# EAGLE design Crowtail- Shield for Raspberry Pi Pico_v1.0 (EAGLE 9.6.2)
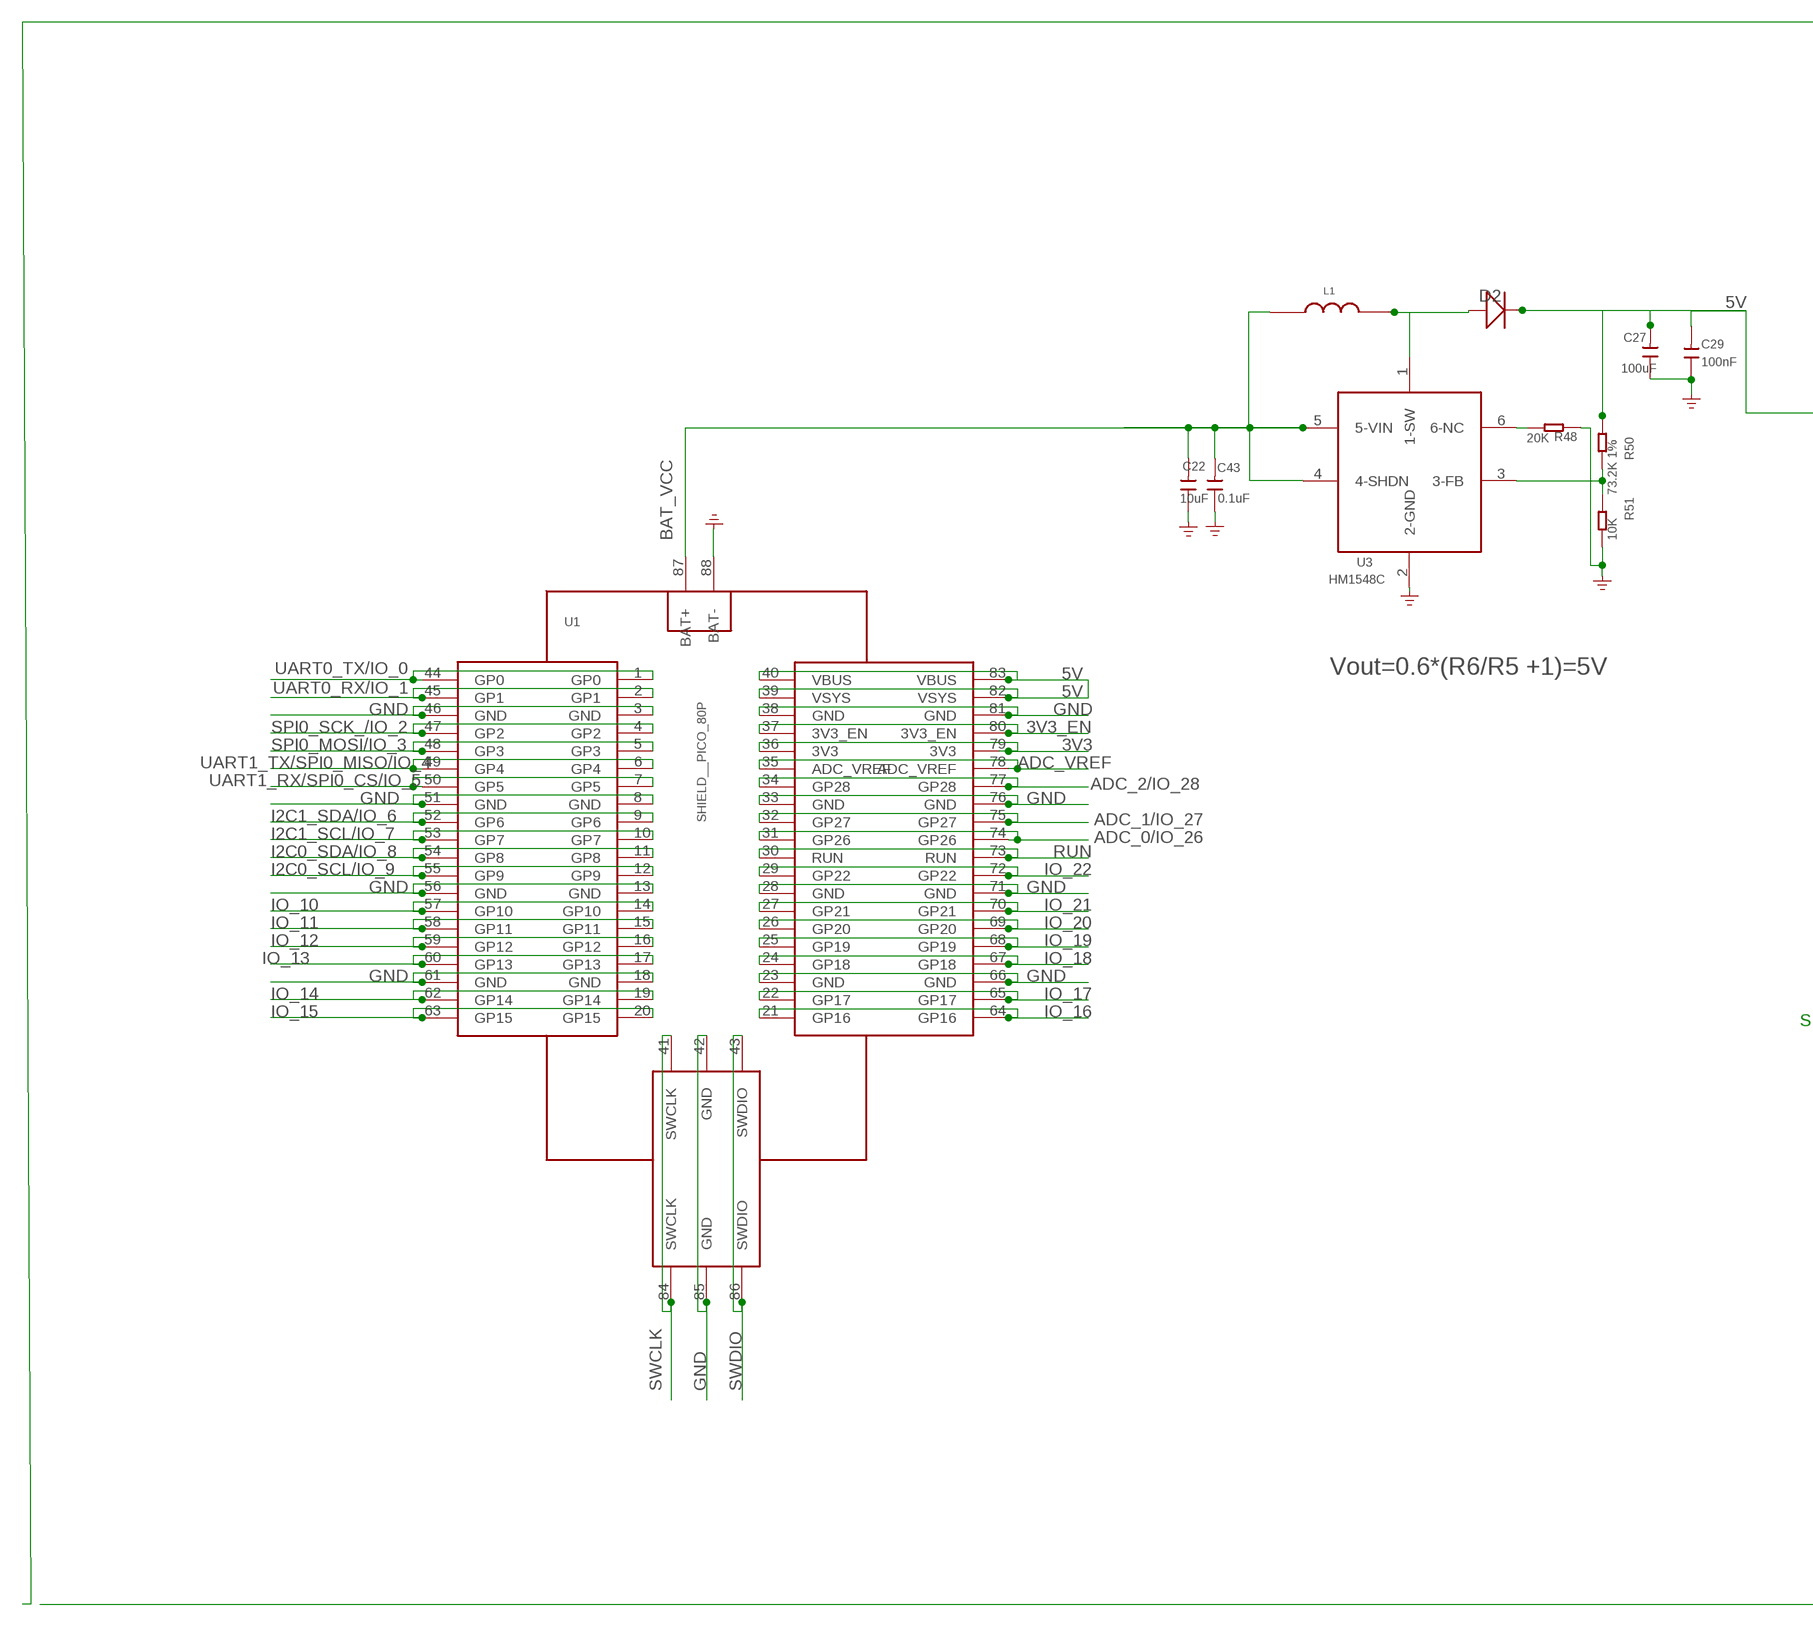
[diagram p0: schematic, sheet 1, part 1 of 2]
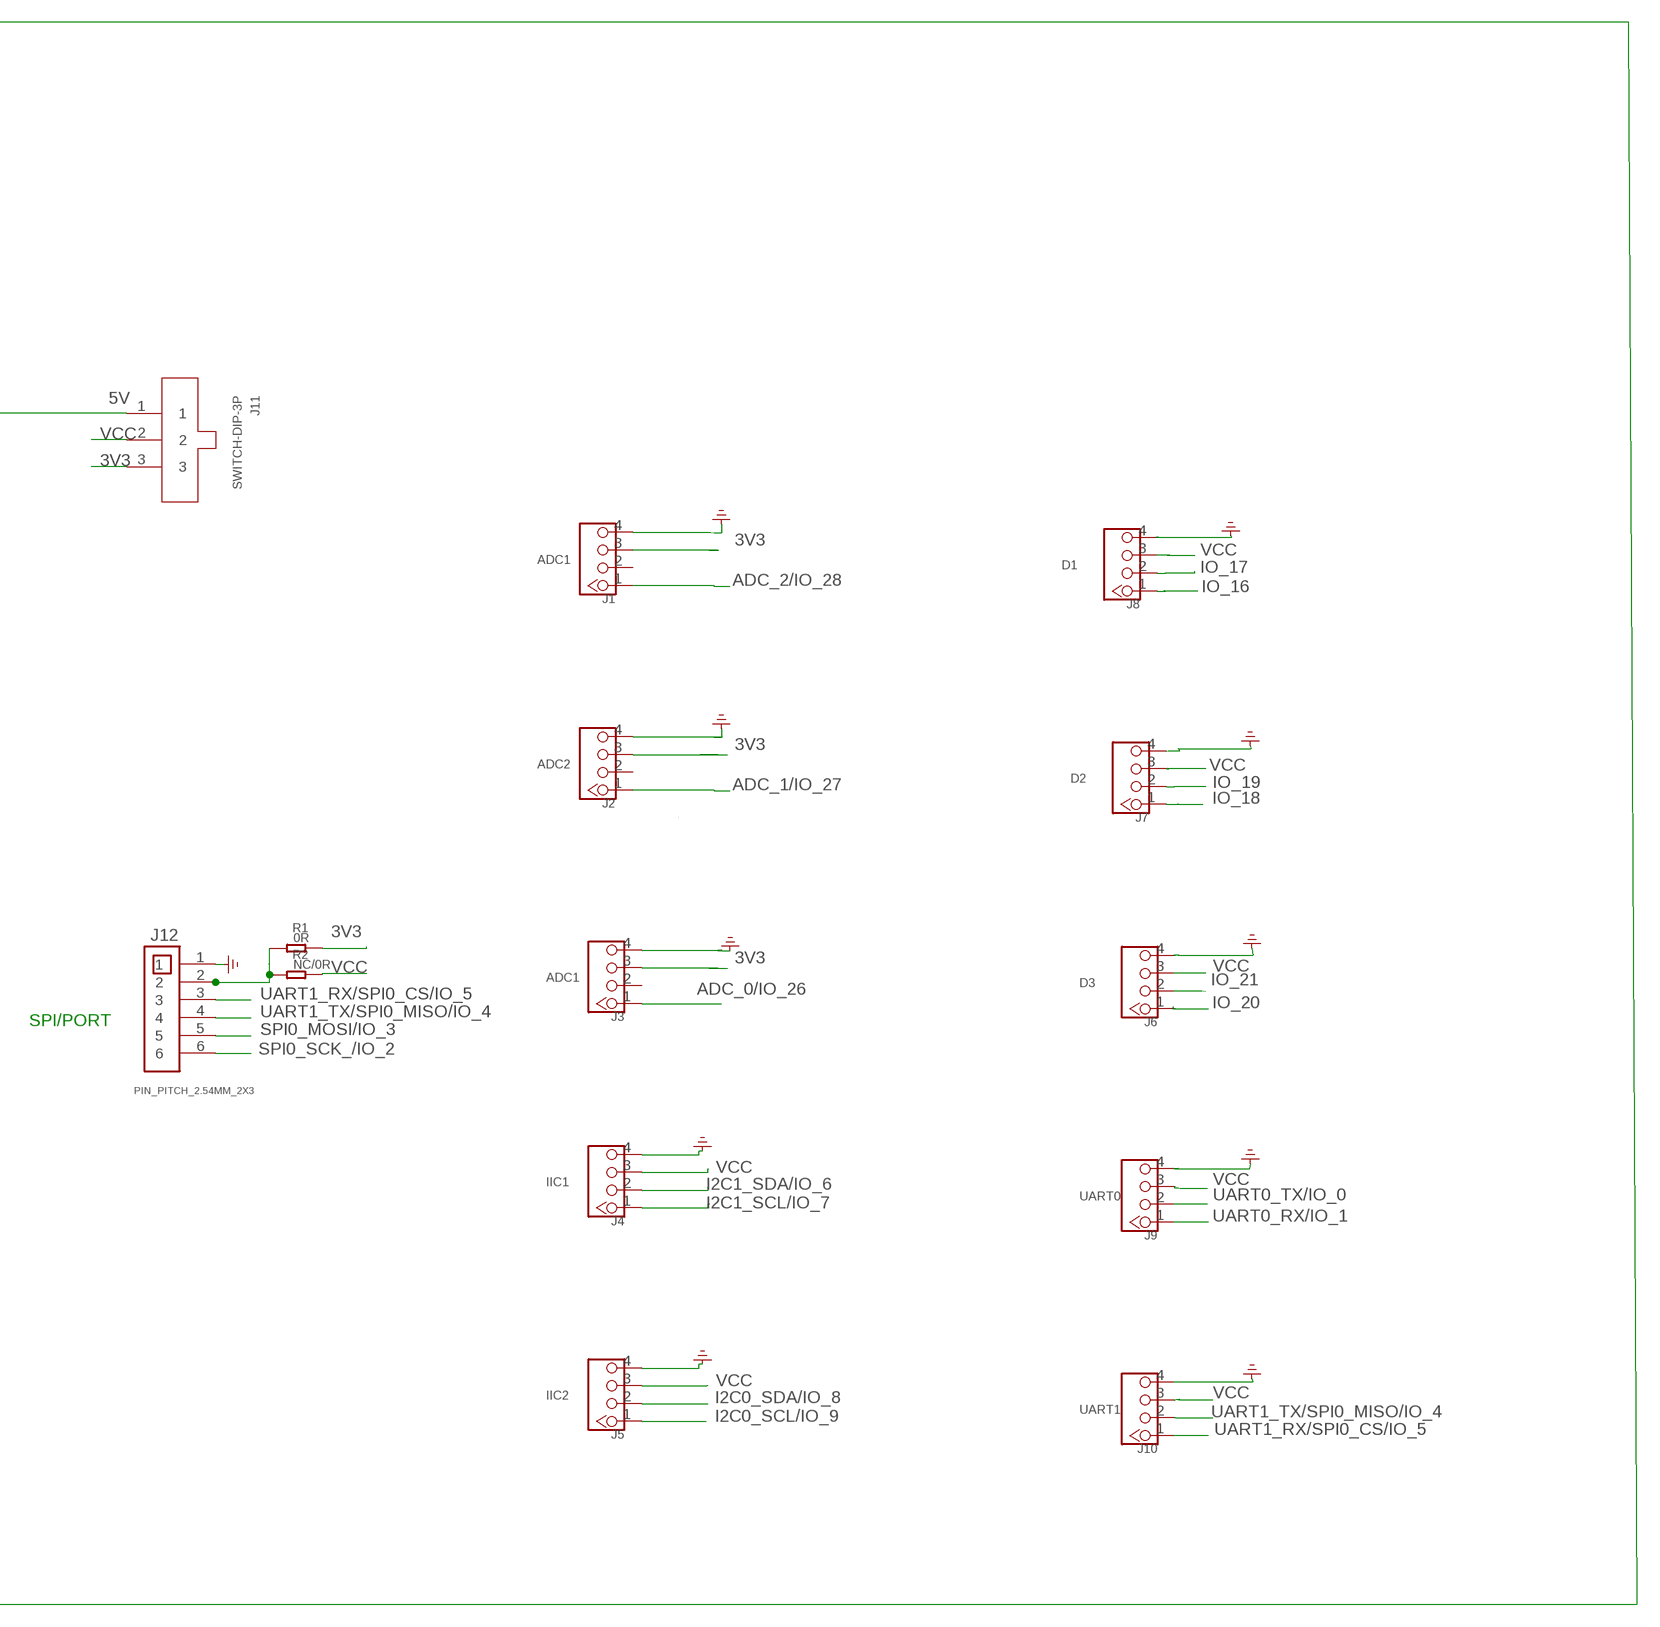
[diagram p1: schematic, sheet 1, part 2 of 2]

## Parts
C22  10uF  C0603  [0603]
C27  100uF  C0805  [0805]
C29  100nF  C0603  [0603]
C43  0.1uF  C0805  [0805]
D2  1N5819/S0D-123  D'1N4148-SMD'  [1206-1]
J1  ADC1  CONNECTOR_TWIG-4P-2.0-2.0  [CONNECTOR_4P-2.0]
J2  ADC2  CONNECTOR_TWIG-4P-2.0-2.0  [CONNECTOR_4P-2.0]
J3  ADC1  CONNECTOR_TWIG-4P-2.0-2.0  [CONNECTOR_4P-2.0]
J4  IIC1  CONNECTOR_TWIG-4P-2.0-2.0  [CONNECTOR_4P-2.0]
J5  IIC2  CONNECTOR_TWIG-4P-2.0-2.0  [CONNECTOR_4P-2.0]
J6  D3  CONNECTOR_TWIG-4P-2.0-2.0  [CONNECTOR_4P-2.0]
J7  D2  CONNECTOR_TWIG-4P-2.0-2.0  [CONNECTOR_4P-2.0]
J8  D1  CONNECTOR_TWIG-4P-2.0-2.0  [CONNECTOR_4P-2.0]
J9  UART0  CONNECTOR_TWIG-4P-2.0-2.0  [CONNECTOR_4P-2.0]
J10  UART1  CONNECTOR_TWIG-4P-2.0-2.0  [CONNECTOR_4P-2.0]
J11  SWITCH-DIP-3P  [SWITCH-DIP-3P]
J12  PIN_PITCH_2.54MM_2X3  [PIN6_PITCH_2.54MM_2X3]
L1  CD32_10uH  CD32_950MA  [CD32]
R1  0R  DISCRETE_R-0603  [DISCRETE_R0603]
R2  NC/0R  DISCRETE_R-0603  [DISCRETE_R0603]
R48  20K  DISCRETE_R-0603  [DISCRETE_R0603]
R50  73.2K 1%  DISCRETE_R-0603  [DISCRETE_R0603]
R51  10K  DISCRETE_R-0603  [DISCRETE_R0603]
U1  SHIELD__PICO_80P  [SHIELD__PICO_80P]
U3  HM1548C  HM1548/SOT23-6  [A_XBJ_SOT23-6]

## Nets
3V1: J12.2 R1.1 R2.1
3V3: J1.3 J2.3 J3.3 J11.3 R1.2 U1.36(3V3) U1.79(3V3)
3V3_EN: U1.37(3V3_EN) U1.80(3V3_EN)
5V: C27.2 C29.2 D2.C(-) J11.1 R50.1 U1.39(VSYS) U1.40(VBUS) U1.82(VSYS) U1.83(VBUS)
ADC_0/IO_26: J3.1 U1.31(GP26) U1.74(GP26)
ADC_1/IO_27: J2.1 U1.32(GP27) U1.75(GP27)
ADC_2/IO_28: J1.1 U1.34(GP28) U1.77(GP28)
ADC_VREF: U1.35(ADC_VREF) U1.78(ADC_VREF)
BAT_VCC: C22.2 C43.2 L1.1 U1.87(BAT+) U3.4(4-SHDN) U3.5(5-VIN)
GND: C22.1 C27.1 C29.1 C43.1 J1.4 J2.4 J3.4 J4.4 J5.4 J6.4 J7.4 J8.4 J9.4 J10.4 J12.1 R48.1 R51.2 U1.3(GND) U1.8(GND) U1.13(GND) U1.18(GND) U1.23(GND) U1.28(GND) U1.33(GND) U1.38(GND) U1.42(GND) U1.46(GND) U1.51(GND) U1.56(GND) U1.61(GND) U1.66(GND) U1.71(GND) U1.76(GND) U1.81(GND) U1.85(GND) U1.88(BAT-) U3.2(2-GND) ; supply symbol labelled GND_POWER
I2C0_SCL/IO_9: J5.1 U1.12(GP9) U1.55(GP9)
I2C0_SDA/IO_8: J5.2 U1.11(GP8) U1.54(GP8)
I2C1_SCL/IO_7: J4.1 U1.10(GP7) U1.53(GP7)
I2C1_SDA/IO_6: J4.2 U1.9(GP6) U1.52(GP6)
IO_10: U1.14(GP10) U1.57(GP10)
IO_11: U1.15(GP11) U1.58(GP11)
IO_12: U1.16(GP12) U1.59(GP12)
IO_13: U1.17(GP13) U1.60(GP13)
IO_14: U1.19(GP14) U1.62(GP14)
IO_15: U1.20(GP15) U1.63(GP15)
IO_16: J8.1 U1.21(GP16) U1.64(GP16)
IO_17: J8.2 U1.22(GP17) U1.65(GP17)
IO_18: J7.1 U1.24(GP18) U1.67(GP18)
IO_19: J7.2 U1.25(GP19) U1.68(GP19)
IO_20: J6.1 U1.26(GP20) U1.69(GP20)
IO_21: J6.2 U1.27(GP21) U1.70(GP21)
IO_22: U1.29(GP22) U1.72(GP22)
N$7: D2.A(+) L1.2 U3.1(1-SW)
N$24: R48.2 U3.6(6-NC)
N$30: R50.2 R51.1 U3.3(3-FB)
RUN: U1.30(RUN) U1.73(RUN)
SPI0_MOSI/IO_3: J12.5 U1.5(GP3) U1.48(GP3)
SPI0_SCK_/IO_2: J12.6 U1.4(GP2) U1.47(GP2)
SWCLK: U1.41(SWCLK) U1.84(SWCLK)
SWDIO: U1.43(SWDIO) U1.86(SWDIO)
UART0_RX/IO_1: J9.1 U1.2(GP1) U1.45(GP1)
UART0_TX/IO_0: J9.2 U1.1(GP0) U1.44(GP0)
UART1_RX/SPI0_CS/IO_5: J10.1 J12.3 U1.7(GP5) U1.50(GP5)
UART1_TX/SPI0_MISO/IO_4: J10.2 J12.4 U1.6(GP4) U1.49(GP4)
VCC: J4.3 J5.3 J6.3 J7.3 J8.3 J9.3 J10.3 J11.2 R2.2
Unconnected: J1.2 J2.2 J3.2

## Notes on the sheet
- Vout=0.6*(R6/R5 +1)=5V
- SPI/PORT

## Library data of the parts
C22 C29 = A_xbj:C0603
C27 C43 = A_xbj:C0805
D2 = Discrete:D*
J1-J10 = Crowtail_Shieldv0_1:CONNECTOR_TWIG-4P-2.0
J11 = Crowtail_Shieldv0_1:SWITCH-DIP-3P
J12 = PIN_PITCH_2.54MM:PIN_PITCH_2.54MM_2X3
L1 = CD54:CD32_950MA
R1 R2 R48 R50 R51 = Crowtail-_LED-V2.0-20190615-01:DISCRETE_R*
U1 = Crowtail_Shieldv0_1:SHIELD__PICO_80P
U3 = CrowBOT-V1.0-20220530库:HM1548/SOT23-6

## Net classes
0 default: width 0.203 mm, drill 0.305 mm, clearance 0.152 mm
3 usbvcc: width 0.203 mm, drill 0.305 mm, clearance 0.203 mm

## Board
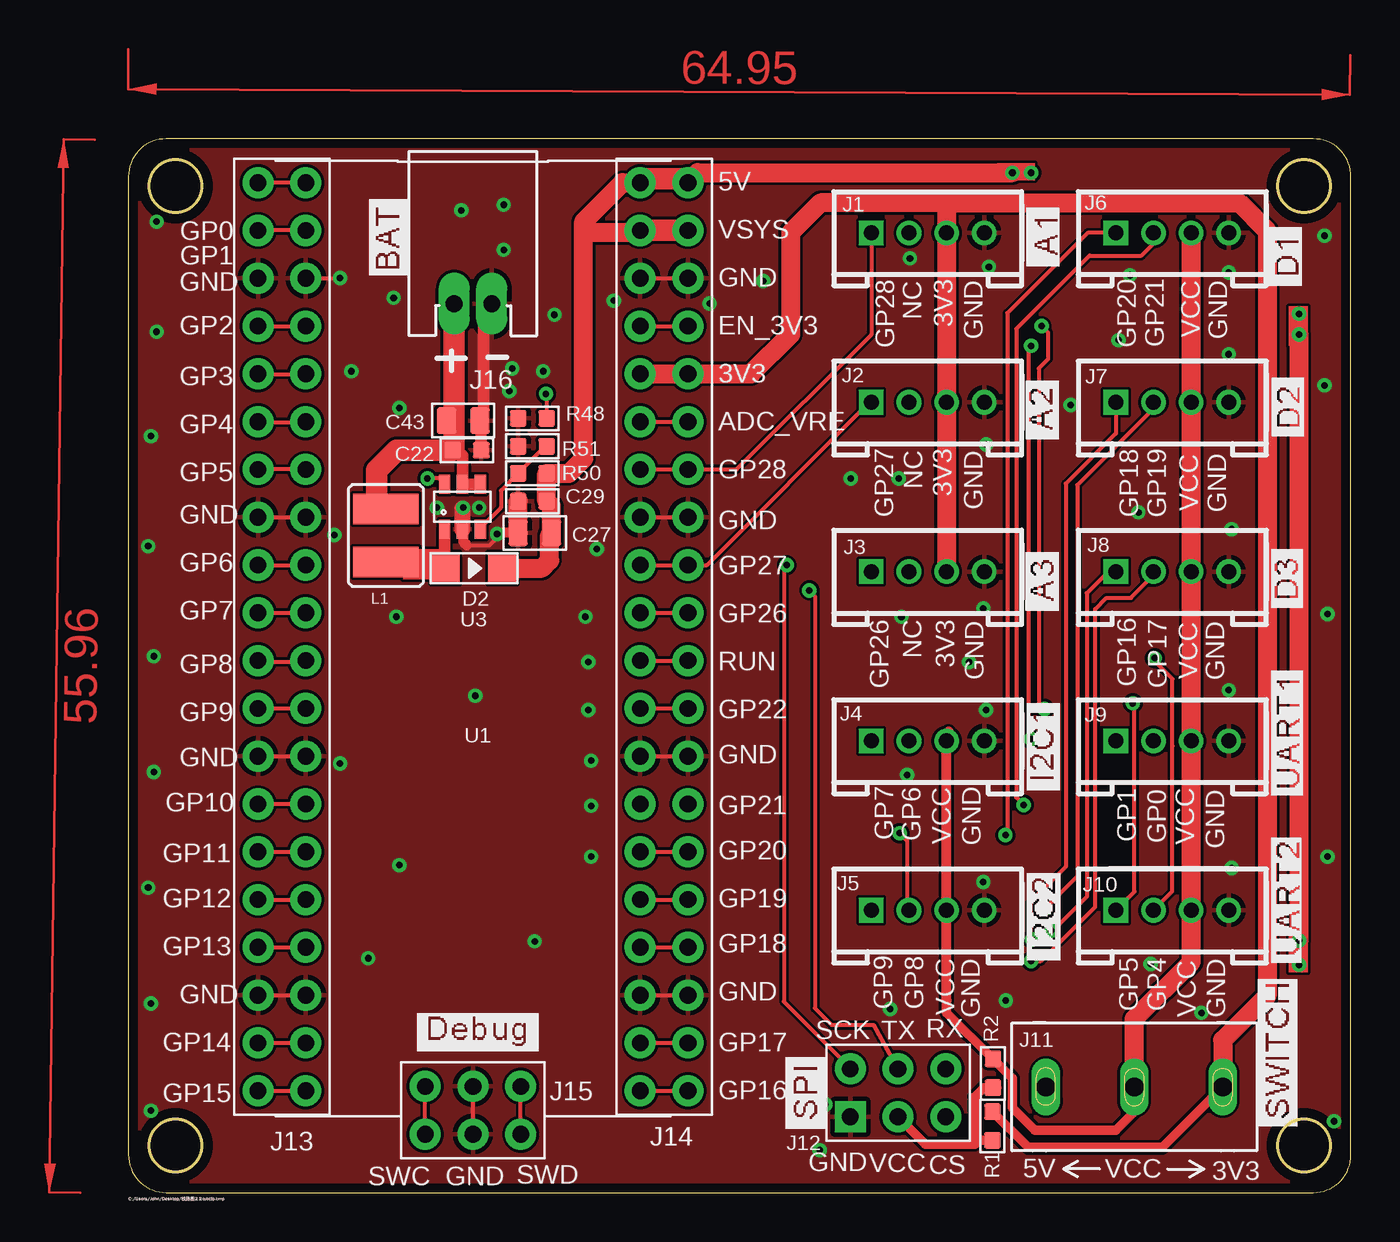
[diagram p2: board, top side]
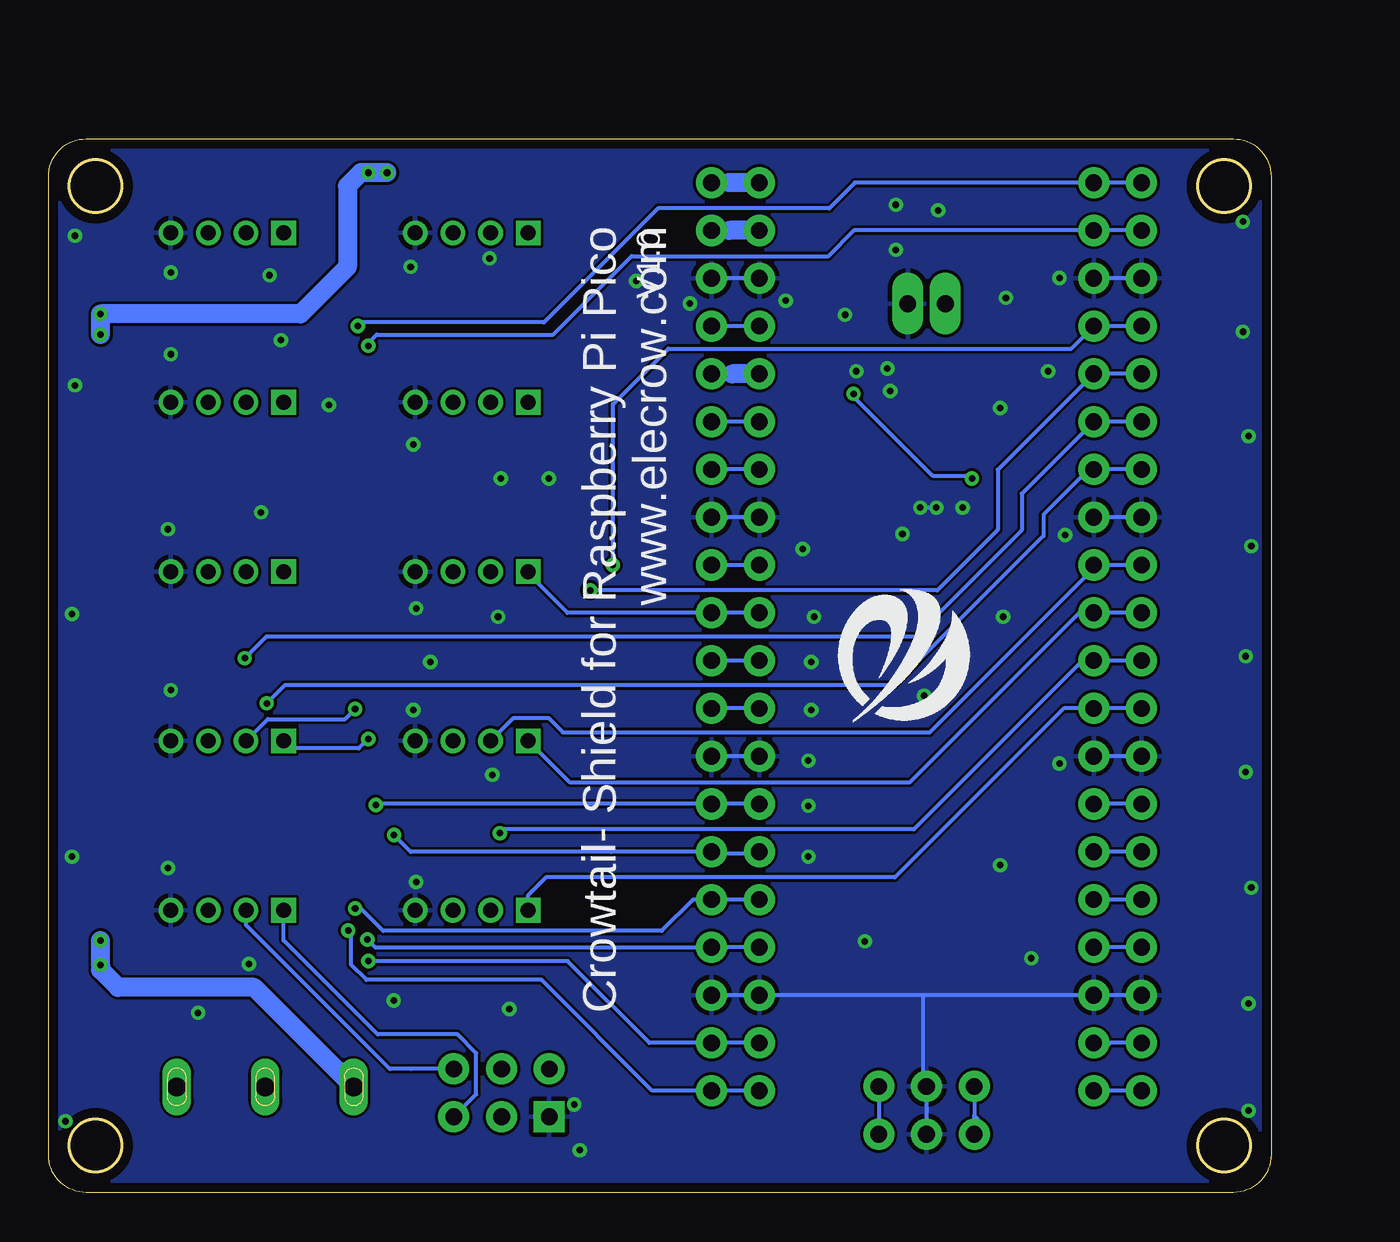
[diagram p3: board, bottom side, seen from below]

Size 65 x 56 mm. Coordinates in mm from the lower left corner, seen from the top.
Outline: 0,54 0,2 arc90 2,0 63,0 arc90 65,2 65,54 arc90 63,56 2,56 arc90 0,54
Outline: circle at 2.5,53.5 radius 1.4
Outline: circle at 2.5,2.5 radius 1.4
Outline: circle at 62.5,53.5 radius 1.4
Outline: circle at 62.5,2.5 radius 1.4
Copper layers (1*16): Top 0.035mm / dielectric 1.5mm / Bottom 0.035mm
Design rules "default *": minimum track width 6mil, minimum drill 0.35mm, track to track 6mil, track to pad 6mil, pad to pad 6mil, via to via 6mil, smd to smd 6mil, copper to edge 20mil, drill to drill 6mil, minimum pad ring 10mil, minimum via ring 8mil, stop-mask expansion 4mil, vias tented up to drill 20mil, thermal gap 10mil

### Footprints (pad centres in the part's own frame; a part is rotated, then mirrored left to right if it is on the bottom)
0603 = smd 0.889 x 0.889: 1 -0.762,0; 2 0.762,0
0805 = smd 1.016 x 1.397: 1 -0.889,0; 2 0.889,0
1206-1 = smd 1.524 x 1.676: A -1.524,0; C 1.524,0
CONNECTOR_4P-2.0 = drill 0.8 pad 1.27 square: 1 -3,0 | drill 0.8 pad 1.27: 2 -1,0; 3 1,0; 4 3,0
SWITCH-DIP-3P = drill 1 long: 1 -4.7,0; 2 0,0; 3 4.7,0
PIN6_PITCH_2.54MM_2X3 = drill 0.889 pad 1.651 square: 1 -1.27,2.54 | drill 0.889 pad 1.651: 2 -1.27,0; 3 -1.27,-2.54; 4 1.27,-2.54; 5 1.27,0; 6 1.27,2.54
CD32 = smd 3.5 x 1.6: 1 0,1.409; 2 0,-1.409
DISCRETE_R0603 = smd 0.889 x 0.889: 1 -0.762,0; 2 0.762,0
SHIELD__PICO_80P = drill 0.889 pad 1.651: 1 -8.89,24.13; 2 -8.89,21.59; 3 -8.89,19.05; 4 -8.89,16.51; 5 -8.89,13.97; 6 -8.89,11.43; 7 -8.89,8.89; 8 -8.89,6.35; 9 -8.89,3.81; 10 -8.89,1.27; 11 -8.89,-1.27; 12 -8.89,-3.81; 13 -8.89,-6.35; 14 -8.89,-8.89; 15 -8.89,-11.43; 16 -8.89,-13.97; 17 -8.89,-16.51; 18 -8.89,-19.05; 19 -8.89,-21.59; 20 -8.89,-24.13; 21 8.89,-24.13; 22 8.89,-21.59; 23 8.89,-19.05; 24 8.89,-16.51; 25 8.89,-13.97; 26 8.89,-11.43; 27 8.89,-8.89; 28 8.89,-6.35; 29 8.89,-3.81; 30 8.89,-1.27; 31 8.89,1.27; 32 8.89,3.81; 33 8.89,6.35; 34 8.89,8.89; 35 8.89,11.43; 36 8.89,13.97; 37 8.89,16.51; 38 8.89,19.05; 39 8.89,21.59; 40 8.89,24.13; 41 -2.54,-23.9; 42 0,-23.9; 43 2.54,-23.9; 44 -11.43,24.13; 45 -11.43,21.59; 46 -11.43,19.05; 47 -11.43,16.51; 48 -11.43,13.97; 49 -11.43,11.43; 50 -11.43,8.89; 51 -11.43,6.35; 52 -11.43,3.81; 53 -11.43,1.27; 54 -11.43,-1.27; 55 -11.43,-3.81; 56 -11.43,-6.35; 57 -11.43,-8.89; 58 -11.43,-11.43; 59 -11.43,-13.97; 60 -11.43,-16.51; 61 -11.43,-19.05; 62 -11.43,-21.59; 63 -11.43,-24.13; 64 11.43,-24.13; 65 11.43,-21.59; 66 11.43,-19.05; 67 11.43,-16.51; 68 11.43,-13.97; 69 11.43,-11.43; 70 11.43,-8.89; 71 11.43,-6.35; 72 11.43,-3.81; 73 11.43,-1.27; 74 11.43,1.27; 75 11.43,3.81; 76 11.43,6.35; 77 11.43,8.89; 78 11.43,11.43; 79 11.43,13.97; 80 11.43,16.51; 81 11.43,19.05; 82 11.43,21.59; 83 11.43,24.13; 84 -2.54,-26.44; 85 0,-26.44; 86 2.54,-26.44 | drill 0.9 pad 1.651 long: 87 -1,17.7; 88 1,17.7
A_XBJ_SOT23-6 = smd 0.6 x 1: 1 -0.95,-1.2; 2 0,-1.2; 3 0.95,-1.2; 4 0.95,1.2; 5 0,1.2; 6 -0.95,1.2

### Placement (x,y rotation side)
C22  18,39.46 180 top
C27  21.61,35.05 0 top
C29  21.48,36.74 0 top
C43  17.8,41.02 180 top
D2  18.37,33.18 0 top
J1  42.5,51 0 top
J2  42.5,42 0 top
J3  42.5,33 0 top
J4  42.5,24 0 top
J5  42.5,15 0 top
J6  55.5,51 0 top
J7  55.5,42 0 top
J8  55.5,33 0 top
J9  55.5,24 0 top
J10  55.5,15 0 top
J11  53.48,5.61 0 top
J12  40.92,5.3 90 top
L1  13.69,34.92 0 top
R1  45.94,3.54 90 top
R2  45.97,6.34 90 top
R48  21.48,41.14 0 top
R50  21.48,38.22 180 top
R51  21.48,39.66 180 top
U1  18.32,29.54 0 top
U3  17.76,36.45 0 top
U$42  [LOGO]  19.31,28.29 90 bottom

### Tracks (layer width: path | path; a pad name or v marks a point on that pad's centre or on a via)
3V1
  Top 0.5: 46.19,5.57 R2.1 45.47,5.57 45,5.1 45,2.77 | R1.1 45,2.77 | J12.2 42.37,2.57 45,2.57 45,2.77
3V3
  Top 0.203: J11.3 58.66,5.61
  Top 0.5: J11.3 54.97,2.4 47.84,2.4 R1.2
  Top 1: U1.36 U1.79 33.11,43.51 35.2,45.6 35.2,51 36.8,52.6 43.5,52.6 | 43.5,52.6 J1.3 J2.3 J3.3 | 43.5,52.6 59.05,52.6 60.55,51.1 60.55,10.47 58.18,8.1 J11.3
  Bottom 0.203: 28.65,43.51 28.79,43.51 28.8,43.5 29.25,43.5 29.26,43.51 U1.79
  Bottom 1: U1.36 28.65,43.51
3V3_EN
  Top 0.203: U1.37 U1.80
  Bottom 0.203: U1.37 28.95,46.05 29.1,45.9
5V  (via drill 0.35)
  Top 1: D2.C 21.98,33.18 22.4,33.6 22.4,34.96 C27.2 22.5,36.49 C29.2 R50.1 23.42,38.22 24.2,39 24.2,51 | 24.2,51 24.2,51.6 26.27,53.67 U1.40 | U1.39 27.08,51 24.2,51 | U1.83 30.28,54.2 v47,54.2 | v62.23,45.6 v62.23,13.4
  Top 1.15: U1.39 U1.82 | U1.40 27.41,53.87 29.55,53.87 U1.83
  Bottom 0.203: 28.83,53.67 28.95,53.55 | 28.8,51.13 29.08,51.13 29.1,51.15
  Bottom 1: U1.40 28.83,53.67 | U1.39 28.8,51.13 | v47,54.2 v48,54.2 48.4,54.2 49.1,53.5 49.1,49.2 51.6,46.7 v62.23,46.7 v62.23,45.6 | J11.1 54.07,10.9 61.3,10.9 62.23,11.83 v62.23,12.1 v62.23,13.4
ADC_0/IO_26
  Top 0.203: U1.31 U1.74
  Bottom 0.203: U1.74 37.41,30.81 39.5,32.9 J3.1 | U1.31 29.04,30.81 29.1,30.75
ADC_1/IO_27
  Top 0.203: U1.32 U1.75 30.75,33.35 39.4,42 J2.1
  Bottom 0.203: U1.32 29.05,33.35 29.1,33.3
ADC_2/IO_28
  Top 0.203: U1.34 U1.77 32.33,38.43 39.5,45.6 J1.1
  Bottom 0.203: U1.34 28.92,38.43 28.95,38.4
ADC_VREF
  Top 0.203: U1.35 U1.78
  Bottom 0.203: U1.35 29.23,40.97 29.25,40.95
BAT_VCC
  Top 0.203: C43.2 17.24,40.69 C22.2 17.48,39.46 17.76,39.18
  Top 0.6: U3.4 U3.5 17.76,39.18
  Top 1.15: U1.87 17.32,39.54 C22.2 14.26,39.46 13.2,38.4 13.2,36.82 L1.1
GND  (via drill 0.35)
  Top 0.203: 18,34.4 19.2,34.4 19.6,34.8 v19.6,35 19.65,35.05 | U1.85 U1.42 | U1.56 U1.13 | U1.61 U1.18 | U1.23 U1.66 | U1.28 U1.71 | U1.33 U1.76 | U1.38 U1.81 | U1.46 7.33,48.15 7.35,48.15 | U1.51 8.66,35.89 8.7,35.85 8.85,35.85 | U1.3 v11.24,48.59 v11.25,48.6
  Top 0.52: C27.1 19.65,35.05 | U3.2 17.8,35.21 17.8,34.6 18,34.4 | 17.76,36.36 v17.8,36.4
  Top 0.6: C22.1 18.76,40.95 C43.1 18.89,41.22 18.89,46.81 U1.88
  Top 0.852: U3.2 17.76,36.36
  Top 1: C27.1 C29.1
  Bottom 0.203: v17.8,36.4 v18.65,36.4 | U1.18 18.5,10.49 | 18.5,10.49 U1.23 28.94,10.49 28.95,10.5 | 18.5,10.49 18.5,5.82 U1.42 18.32,3.62 18.3,3.6 | U1.46 U1.3 | U1.51 U1.8 | U1.56 9.84,23.19 10.05,23.4 9.82,23.62 | U1.61 8.54,10.49 8.55,10.5 | U1.38 29.09,48.59 29.1,48.6 | U1.33 28.91,35.89 29.1,35.7 | U1.28 29.04,23.19 29.1,23.25
  other vias: 16.4,36.4 1.5,51.6 1.5,45.75 1.2,40.2 1.05,34.35 1.35,28.5 1.35,22.35 1.05,16.2 1.2,10.05 1.2,4.35 10.95,34.95 11.25,22.8 14.4,17.4 21.6,13.35 12.75,12.45 24.6,17.85 24.6,20.55 24.6,22.95 24.45,25.65 24.45,28.2 18.45,26.4 14.25,30.6 24.3,30.6 24.9,34.2 14.1,47.55 19.95,50.1 19.95,52.5 17.7,52.2 20.4,43.8 20.25,42.6 22.65,46.65 22.05,43.65 11.85,43.65 14.4,41.7 30.9,47.25 33.75,48.45 25.8,47.4 45.6,39.75 38.4,37.95 40.95,37.95 41.55,49.65 45.75,49.2 45.45,31.05 41.1,30.6 45.6,25.65 41.4,22.2 45.45,16.5 37.06,4.68 36.75,2.25 40.5,9.75 46.65,10.2 57.05,9.55 54.35,12.15 58.65,17.25 58.5,26.7 58.65,35.25 53.7,36.15 44.7,28.2 58.5,44.55 52.65,45.3 50.1,41.85 58.5,48.9 53.25,48.75 63.6,50.85 63.6,42.9 63.75,30.75 63.75,17.85 64.1,3.79
  pour Top: -0.45,55.95 -0.45,-0.3 -0.15,-0.6 63.75,-0.6 65.25,0.9 65.25,55.05 65.1,55.2 64.2,56.1 -0.3,56.1
  pour Bottom: -0.3,56.25 -0.3,0.15 0.6,-0.75 63.6,-0.75 65.25,0.9 65.25,54.45 64.2,55.5
I2C0_SCL/IO_9
  Top 0.203: U1.55 8.63,25.73 8.7,25.8
  Bottom 0.203: J5.1 39.5,15.8 38.55,16.75 20,16.75 11.02,25.73 U1.12 U1.55
I2C0_SDA/IO_8  (via drill 0.35)
  Top 0.203: v41,19.1 41.4,18.7 41.4,15.1 J5.2 | U1.54 6.96,28.2 8.85,28.2
  Bottom 0.203: v41,19.1 40.8,19.3 19,19.3 10.03,28.27 U1.11 U1.54
I2C1_SCL/IO_7
  Top 0.203: U1.53 U1.10
  Bottom 0.203: J4.1 37.31,21.81 19.19,21.81 10.19,30.81 9.75,30.81 U1.10 U1.53
I2C1_SDA/IO_6
  Top 0.203: U1.52 U1.9
  Bottom 0.203: 9.43,33.17 18.15,24.45 37.65,24.45 38.4,25.2 40.3,25.2 J4.2 | U1.9 9.43,33.17 | U1.52 9.25,33.35 9.43,33.17
IO_10
  Top 0.203: U1.57 8.6,20.65 8.7,20.55
  Bottom 0.203: U1.57 U1.14
IO_11
  Top 0.203: U1.58 8.66,18.11 8.7,18.15
  Bottom 0.203: U1.58 U1.15
IO_12
  Top 0.203: U1.59 U1.16
  Bottom 0.203: U1.59 8.58,15.57 8.7,15.45 8.78,15.53
IO_13
  Top 0.203: U1.60 U1.17
  Bottom 0.203: U1.60 8.68,13.03 8.7,13.05
IO_14
  Top 0.203: U1.62 U1.19
  Bottom 0.203: U1.62 8.55,7.95 8.7,7.8
IO_15
  Top 0.203: U1.63 U1.20
  Bottom 0.203: U1.63 8.69,5.41 8.7,5.4
IO_16  (via drill 0.35)
  Top 0.203: U1.21 U1.64 | v49.07,13.93 49.17,13.93 50.95,15.71 50.95,31.85 52.1,33 J8.1
  Bottom 0.203: U1.64 32.91,5.41 38.8,11.3 48.1,11.3 48.9,12.1 48.9,13.76 v49.07,13.93 | U1.21 29.1,5.4
IO_17  (via drill 0.35)
  Top 0.203: U1.22 U1.65 | v48,12.3 48.5,12.3 51.4,15.2 51.4,31 52,31.6 53.3,31.6 54.6,32.9 J8.2
  Bottom 0.203: U1.65 33.05,7.95 37.4,12.3 v48,12.3 47.7,12.3 | U1.22 29.25,7.95
IO_18  (via drill 0.35)
  Top 0.203: U1.24 30.17,13.03 30.2,13 | J7.1 52.5,40.35 49.83,37.68 49.83,17.33 47.97,15.46 47.97,13.53 v48.05,13.45
  Bottom 0.203: v48.05,13.45 47.63,13.03 U1.67 28.97,13.03 28.95,13.05 28.93,13.03 U1.24
IO_19  (via drill 0.35)
  Top 0.203: U1.25 U1.68 | v48.7,15.1 48.75,15.1 50.45,16.8 50.45,37.6 54.5,41.65 J7.2
  Bottom 0.203: U1.68 30.73,15.57 32.4,13.9 47.2,13.9 48.4,15.1 v48.7,15.1 | U1.25 29.07,15.57 29.1,15.6
IO_20  (via drill 0.35)
  Top 0.203: U1.26 U1.69 | U1.69 29.89,18.11 30.2,17.8 30.06,17.8 U1.69 | J6.1 51,51 46.73,46.73 46.73,19.1 v46.63,19
  Bottom 0.203: U1.69 35.09,18.11 45.74,18.11 v46.63,19 | U1.26 27.32,18 29.1,18
IO_21  (via drill 0.35)
  Top 0.203: v47.6,20.6 47.2,21 47.2,45.9 51.09,49.79 53.86,49.79 54.5,50.43 J6.2
  Bottom 0.203: v47.6,20.6 47.55,20.65 U1.70 U1.27
IO_22
  Top 0.203: U1.29 U1.72
  Bottom 0.203: U1.29 29.18,25.73 29.25,25.8
N$7
  Top 0.203: D2.A 16.81,33.22 U3.1
  Top 0.6: L1.2 16.09,33.51 16.6,33 16.81,33.21 U3.1
N$24  (via drill 0.35)
  Top 0.203: U3.6 16.51,37.95 v15.9,37.95 | v22.2,42.45 22.24,42.41 R48.2
  Bottom 0.203: v15.9,37.95 16.05,38.1 18,38.1 22.2,42.3 v22.2,42.45
N$30
  Top 0.203: R51.1 22.16,39.66 R50.2 19.8,37.3 19.8,36.4 18.71,35.31 U3.3
RUN
  Top 0.203: U1.30 U1.73
  Bottom 0.203: U1.30 29.03,28.27 29.1,28.2
SPI0_MOSI/IO_3  (via drill 0.35)
  Top 0.203: v36.2,32 36.5,31.7 36.5,9.8 37.4,8.9 39.63,8.9 J12.5 | U1.48 8.85,43.5
  Bottom 0.203: v36.2,32 17.75,32 14.53,35.23 14.53,38.41 U1.5 U1.48
SPI0_SCK_/IO_2  (via drill 0.35)
  Top 0.203: v35,33.35 34.85,33.2 34.85,10.15 38.37,6.63 J12.6 | 9.6,45.45 9,46.05 U1.47
  Bottom 0.203: v35,33.35 35,41.9 32.05,44.85 10.63,44.85 U1.4 U1.47
SWCLK
  Top 0.203: U1.84 U1.41
  Bottom 0.203: U1.41 15.78,4.08 | 15.78,4.08 15.6,3.9 | U1.84 15.78,4.08
SWDIO
  Top 0.203: U1.86 U1.43
  Bottom 0.203: U1.43 20.86,3.91 20.7,3.75
UART0_RX/IO_1  (via drill 0.35)
  Top 0.203: U1.2 U1.45 | v48,45 47.85,44.85 47.85,24.25 v48,24.1
  Bottom 0.203: v48,24.1 48.5,23.6 52.2,23.6 52.5,23.9 J9.1 | v48,45 48,45.15 47.55,45.6 38.17,45.6 34,49.77 23.53,49.77 22.17,51.13 U1.2 U1.45
UART0_TX/IO_0  (via drill 0.35)
  Top 0.203: U1.1 U1.44 | v48.7,25.7 48.4,26 48.4,43.8 48.9,44.3 48.9,45.7 v48.55,46.05
  Bottom 0.203: v48.7,25.7 49.24,25.16 53.34,25.16 J9.2 | v48.55,46.05 48.35,46.25 38.66,46.25 32.6,52.31 23.49,52.31 22.13,53.67 U1.1 U1.44
UART1_RX/SPI0_CS/IO_5  (via drill 0.35)
  Top 0.203: U1.7 U1.50 | v53.4,26 53.49,25.91 53.49,15.99 J10.1
  Bottom 0.203: v53.4,26 52.45,26.95 20.05,26.95 12.1,34.9 12.1,36.01 9.68,38.43 U1.7 U1.50 | J12.3 42.27,5.22 42.27,7.41 43.25,8.4 47.5,8.4 52.5,13.4 J10.1
UART1_TX/SPI0_MISO/IO_4  (via drill 0.35)
  Top 0.203: v54.57,28.4 54.57,28.24 55.51,27.3 55.51,23.72 55.5,23.72 55.5,16 J10.2 | U1.49 6.91,40.95 8.85,40.95
  Bottom 0.203: J10.2 54.5,14.21 46.86,6.57 45.7,6.57 J12.4 | v54.57,28.4 53.42,29.55 18.9,29.55 13.25,35.2 13.25,37.15 U1.6 U1.49
VCC
  Top 0.5: 53.48,8.9 J11.2 53.48,4.28 52.5,3.3 48.2,3.3 47,4.5 47,6.07 R2.2 43.5,9.56 43.5,10.2
  Top 0.52: J4.3 J5.3 43.5,10.2 | J4.3 43.5,24.4 43.6,24.5 43.6,24.1 J4.3
  Top 1: J6.3 J7.3 J8.3 J9.3 J10.3 56.5,12.24 53.48,9.22 J11.2
(copper drawn outside any net)
  shapes: Top area x6

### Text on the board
tPlace: 5V | GP0 | VSYS | GP1 | GP28 | 3V3 | GP20 | GP21 | GND | GND | NC | GND | VCC | GND | GP2 | EN_3V3 | GP3 | 3V3 | GP4 | ADC_VRE | GP27 | 3V3 | GP18 | GP19 | NC | GND | VCC | GND | GP5 | GP28 | GND | GND | GP6 | GP27 | GP16 | GP7 | GP26 | GP26 | NC | 3V3 | GND | GP17 | VCC | GND | GP8 | RUN | GP9 | GP22 | GND | GND | GP7 | GP6 | VCC | GND | GP1 | VCC | GP0 | GND | GP10 | GP21 | GP11 | GP20 | GP12 | GP19 | GP13 | GP18 | GP9 | GP8 | VCC | GND | GP5 | GP4 | VCC | GND | GND | GND | SCK | TX | RX | GP14 | GP17 | GP15 | GP16 | GND | VCC | CS | VCC | SWC | GND | SWD | 5V | 3V3 | C:/Users/John/Desktop/线路图2 luo.bmp | C:/Users/John/Desktop/线路图2.2 luo(1).bmp | C:/Users/John/Desktop/线路图2.2 luo(2).bmp
bPlace: V1.0 | Crowtail- Shield for Raspberry Pi Pico / www.elecrow.com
